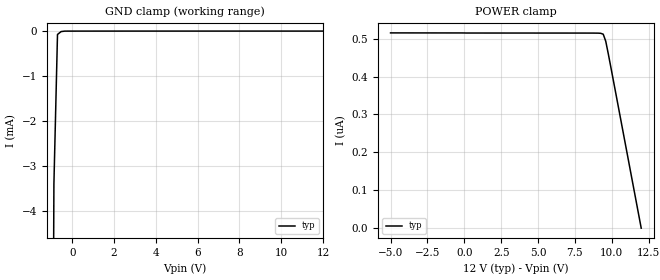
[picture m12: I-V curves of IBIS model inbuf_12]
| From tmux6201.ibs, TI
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| inbuf_12
[Model]   inbuf_12
Model_type   Input
Vinl = 0.8
Vinh = 1.3
|   typ   min   max
C_comp   4.014581e-13   NA   NA
[Voltage Range]   12   NA   NA
[Temperature Range]   27   NA   NA
[Power Clamp Reference]   12   NA   NA
[GND Clamp Reference]   0   NA   NA
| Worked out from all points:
|   GND clamp passes 1 mA (typ) near -0.75 V on its own axis
[GND Clamp]
|   Voltage   I(typ)   I(min)   I(max)
-5V       -1.213A    NA         NA
-1.051V   -21.74mA   NA         NA
-878.8mV  -3.404mA   NA         NA
-707.1mV  -74.78uA   NA         NA
-535.4mV  -10.83uA   NA         NA
12V       514.9nA    NA         NA
[POWER Clamp]
|   Voltage   I(typ)   I(min)   I(max)
-5V       515.1nA    NA         NA
8.737V    514.5nA    NA         NA
9.253V    514nA      NA         NA
9.424V    511.6nA    NA         NA
9.596V    492.8nA    NA         NA
9.768V    459.7nA    NA         NA
12V       -74.91pA   NA         NA
